|Texas Instruments Incorporated
|IWR1843 Single-Chip 60- to 64-GHz mmWave Sensor
[IBIS Ver]   4.1
[File name]   iwr1843.ibs
[Date]   10/12/2018
[File Rev]   1.0
[Source]
| Texas Instruments Incorporated.
| Analog-eLab Design Center, HPA
| 12500 TI Blvd
| Dallas, TX -75243
[Notes]   Revision History:
| Rev 1.0: 10/12/2018
| - Initial version of the model
| - C_comp although listed in numerical order of value are
|   obtained from varying PVT conditions. For PVT conditions for
|   each specific value refer the buffer description under
|   respective [Model]. IBIS model user is responsible for using
|   appropriate C_comp to simulate for Signal Integrity.
| Rev 1.1  9/9/2019
|  - Added missing package model keyword
|  - Removed redundant references
[Disclaimer]
| This model is designed as an aid for customers of Texas Instruments.
| TI and its licensors and suppliers make no warranties, either expressed
| or implied, with respect to this  model, including the warranties of
| merchantability or fitness for a particular purpose. The model is
| provided solely on an "as is" basis. The entire risk as to its quality
| and performance is with the customer.
| This model is subject to change without notice. Texas Instruments
| Incorporated is not responsible for updating this model.
[Copyright]
(C) Copyright 2018 Texas Instruments Incorporated.All rights reserved.
|  Component IWR1843QGABL
[Component]   IWR1843QGABL
[Manufacturer]   Texas Instruments
[Package]   |161 FCBGA -ABL0161 package
|  variable   typ   min   max
R_pkg   0.05   0.04   0.06
L_pkg   1.0nH   0.8nH   1.2nH
C_pkg   0.2pF   0.16pF   0.24pF
[Pin]   signal_name   model_name   R_pin   L_pin   C_pin
 A1   VSSA   GND   NA   NA   NA
 A2   VOUT_PA   NC   NA   NA   NA
 A3   VSSA   GND   NA   NA   NA
 A5   VSSA   GND   NA   NA   NA
 A7   VSSA   GND   NA   NA   NA
 A9   VSSA   GND   NA   NA   NA
 A10   VOUT_14APLL   NC   NA   NA   NA
 A13   VSSA   GND   NA   NA   NA
 A14   OSC_CLKOUT   NC   NA   NA   NA
 A15   VSSA   GND   NA   NA   NA
 B1   VSSA   GND   NA   NA   NA
 B2   VOUT_PA   NC   NA   NA   NA
 B3   VSSA   GND   NA   NA   NA
 B4   TX1   NC   NA   NA   NA
 B5   VSSA   GND   NA   NA   NA
 B6   TX2   NC   NA   NA   NA
 B7   VSSA   GND   NA   NA   NA
 B8   TX3   NC   NA   NA   NA
 B9   VSSA   GND   NA   NA   NA
 B10   VBGAP   NC   NA   NA   NA
 B11   VIN_18CLK   POWER   NA   NA   NA
 B12   VIN_18VCO   POWER   NA   NA   NA
 B13   VOUT_14SYNTH   NC   NA   NA   NA
 B14   VSSA   GND   NA   NA   NA
 B15   CLKP   NC   NA   NA   NA
 C1   VSSA   GND   NA   NA   NA
 C2   VIN_13RF2   POWER   NA   NA   NA
 C3   VSSA   GND   NA   NA   NA
 C4   VSSA   GND   NA   NA   NA
 C5   VSSA   GND   NA   NA   NA
 C6   VSSA   GND   NA   NA   NA
 C7   VSSA   GND   NA   NA   NA
 C8   VSSA   GND   NA   NA   NA
 C9   VSSA   GND   NA   NA   NA
 C13   GPADC5   NC   NA   NA   NA
 C14   VSSA   GND   NA   NA   NA
 C15   CLKM   NC   NA   NA   NA
 D2   VIN_13RF2   POWER   NA   NA   NA
 D13   SPIA_MOSI   IO1   NA   NA   NA
 D14   GPADC6   NC   NA   NA   NA
 D15   VIOIN_18DIFF   POWER   NA   NA   NA
 E1   VSSA   GND   NA   NA   NA
 E2   VSSA   GND   NA   NA   NA
 E3   VSSA   GND   NA   NA   NA
 E5   VSS   GND   NA   NA   NA
 E6   VSS   GND   NA   NA   NA
 E8   VSS   GND   NA   NA   NA
 E10   VSS   GND   NA   NA   NA
 E11   VSS   GND   NA   NA   NA
 E13   SPIA_CLK   IO1   NA   NA   NA
 E14   SPIA_MISO   IO1   NA   NA   NA
 E15   SPIA_CS_N   IO1   NA   NA   NA
 F2   RX4   NC   NA   NA   NA
 F3   VSSA   GND   NA   NA   NA
 F5   VIN_18BB   POWER   NA   NA   NA
 F9   VSS   GND   NA   NA   NA
 F11   VSS   GND   NA   NA   NA
 F13   SPIB_MOSI   IO1   NA   NA   NA
 F14   SPIB_CLK   IO1   NA   NA   NA
 F15   VIOIN   POWER   NA   NA   NA
 G1   VSSA   GND   NA   NA   NA
 G2   VSSA   GND   NA   NA   NA
 G3   VSSA   GND   NA   NA   NA
 G5   VIN_13RF1   POWER   NA   NA   NA
 G6   VSS   GND   NA   NA   NA
 G7   VSS   GND   NA   NA   NA
 G8   VSS   GND   NA   NA   NA
 G10   VSS   GND   NA   NA   NA
 G13   SYNC_OUT   IO2   NA   NA   NA
 G14   SPIB_MISO   IO1   NA   NA   NA
 G15   VIN_SRAM   POWER   NA   NA   NA
 H2   RX3   NC   NA   NA   NA
 H3   VSSA   GND   NA   NA   NA
 H5   VIN_13RF1   POWER   NA   NA   NA
 H7   VSS   GND   NA   NA   NA
 H9   VSS   GND   NA   NA   NA
 H11   VSS   GND   NA   NA   NA
 H13   GPIO_0   IO1   NA   NA   NA
 H14   SPIB_CS_N   IO1   NA   NA   NA
 H15   VDDIN   POWER   NA   NA   NA
 J1   VSSA   GND   NA   NA   NA
 J2   VSSA   GND   NA   NA   NA
 J3   VSSA   GND   NA   NA   NA
 J5   VIN_13RF1   POWER   NA   NA   NA
 J6   VSS   GND   NA   NA   NA
 J7   VSS   GND   NA   NA   NA
 J8   VSS   GND   NA   NA   NA
 J10   VSS   GND   NA   NA   NA
 J13   GPIO_1   IO1   NA   NA   NA
 J14   LVDS_TXP[0]   ODF   NA   NA   NA
 J15   LVDS_TXM[0]   ODF   NA   NA   NA
 K2   RX2   NC   NA   NA   NA
 K3   VSSA   GND   NA   NA   NA
 K5   VIN_18BB   POWER   NA   NA   NA
 K7   VSS   GND   NA   NA   NA
 K8   VSS   GND   NA   NA   NA
 K9   VSS   GND   NA   NA   NA
 K10   VSS   GND   NA   NA   NA
 K11   VSS   GND   NA   NA   NA
 K13   GPIO_2   IO2   NA   NA   NA
 K14   LVDS_TXP[1]   ODF   NA   NA   NA
 K15   LVDS_TXM[1]   ODF   NA   NA   NA
 L1   VSSA   GND   NA   NA   NA
 L2   VSSA   GND   NA   NA   NA
 L3   VSSA   GND   NA   NA   NA
 L5   VSS   GND   NA   NA   NA
 L6   VSS   GND   NA   NA   NA
 L8   VSS   GND   NA   NA   NA
 L10   VSS   GND   NA   NA   NA
 L13   VPP   POWER   NA   NA   NA
 L14   LVDS_CLKP   ODF   NA   NA   NA
 L15   LVDS_CLKM   ODF   NA   NA   NA
 M2   RX1   NC   NA   NA   NA
 M3   VSSA   GND   NA   NA   NA
 M14   LVDS_FRCLKP   ODF   NA   NA   NA
 M15   LVDS_FRCLKM   ODF   NA   NA   NA
 N1   VSSA   GND   NA   NA   NA
 N2   VSSA   GND   NA   NA   NA
 N3   VSSA   GND   NA   NA   NA
 N4   RS232_RX   IO1   NA   NA   NA
 N5   RS232_TX   IO1   NA   NA   NA
 N6   NERROR_OUT   IOOD   NA   NA   NA
 N7   NERROR_IN   IOOD   NA   NA   NA
 N8   MCU_CLKOUT   IO1   NA   NA   NA
 N9   WARM_RESET   IOOD   NA   NA   NA
 N10   TMS   IO2   NA   NA   NA
 N11   VDDIN   POWER   NA   NA   NA
 N12   QSPI[1]   IO1   NA   NA   NA
 N13   TDO   IO2   NA   NA   NA
 N14   DMM_SYNC   IO1   NA   NA   NA
 N15   GPIO_47   IO1   NA   NA   NA
 P1   GPADC1   NC   NA   NA   NA
 P2   GPADC2   NC   NA   NA   NA
 P3   GPADC3   NC   NA   NA   NA
 P4   SYNC_IN   IO2   NA   NA   NA
 P5   GPIO_32   IO1   NA   NA   NA
 P6   GPIO_34   IO1   NA   NA   NA
 P7   GPIO_36   IO1   NA   NA   NA
 P8   GPIO_38   IO1   NA   NA   NA
 P9   PMIC_CLKOUT   IO2   NA   NA   NA
 P10   TCK   IO2   NA   NA   NA
 P11   QSPI_CS_N   IO1   NA   NA   NA
 P12   QSPI[3]   IO1   NA   NA   NA
 P13   SPI_HOST_INTR   NC   NA   NA   NA
 P14   VNWA   POWER   NA   NA   NA
 P15   VDDIN   POWER   NA   NA   NA
 R1   VSSA   GND   NA   NA   NA
 R2   GPADC4   NC   NA   NA   NA
 R3   NRESET   NC   NA   NA   NA
 R4   GPIO_31   IO1   NA   NA   NA
 R5   GPIO_33   IO1   NA   NA   NA
 R6   VDDIN   POWER   NA   NA   NA
 R7   GPIO_35   IO1   NA   NA   NA
 R8   GPIO_37   IO1   NA   NA   NA
 R9   VIOIN_18   POWER   NA   NA   NA
 R10   VIOIN   POWER   NA   NA   NA
 R11   TDI   IO2   NA   NA   NA
 R12   QSPI_CLK   IO1   NA   NA   NA
 R13   QSPI[0]   IO2   NA   NA   NA
 R14   QSPI[2]   IO2   NA   NA   NA
 R15   VSS   GND   NA   NA   NA
[Diff Pin]  inv_pin  vdiff  tdelay_typ  tdelay_min  tdelay_max
   J14   J15   0.1   NA   NA   NA
   K14   K15   0.1   NA   NA   NA
   L14   L15   0.1   NA   NA   NA
   M14   M15   0.1   NA   NA   NA
[Package Model]  IWR1843QGABL
| Model IOOD
[Model Selector] IOOD
|SC1 IS A SLEW RATE CONTROL PIN
|5% SUPPLY VARIATION MODES WITH 1.8V NOM SUPPLY
IOOD_V_PUPDOFF_5P_SC1_1P8  Cell operated at 1.8(nom)
|IOOD_V_PUPDOFF_5P_SC1_1P8; BUFFER WITH WEAK PULUP/PULLDOWN OFF AT 5% SUPPLY
|VARIATION WITH SC1=1 MEANING SLOW MODE OF OPERATION
IOOD_V_PD_ON_5P_!SC1_1P8  Cell operated at 1.8(nom)
|IOOD_V_PD_ON_5P_!SC1_1P8; BUFFER WITH WEAK_PULLDOWN_ON AT 5% SUPPLY
|VARIATION WITH SC1=0 MEANING FAST MODE OF OPERATION
IOOD_V_PD_ON_5P_SC1_1P8  Cell operated at 1.8(nom)
|IOOD_V_PD_ON_5P_SC1_1P8; BUFFER WITH WEAK_PULLDOWN_ON AT 5% SUPPLY
|VARIATION WITH SC1=1 MEANING SLOW MODE OF OPERATION
IOOD_V_PU_ON_5P_!SC1_1P8  Cell operated at 1.8(nom)
|IOOD_V_PU_ON_5P_!SC1_1P8; BUFFER WITH WEAK_PULLUP_ON AT 5% SUPPLY
|VARIATION WITH SC1=0 MEANING FAST MODE OF OPERATION
IOOD_V_PUPDOFF_5P_!SC1_1P8  Cell operated at 1.8(nom)
|IOOD_V_PUPDOFF_5P_!SC1_1P8; BUFFER WITH WEAK PULUP/PULLDOWN OFF AT 5% SUPPLY
|VARIATION WITH SC1=0 MEANING FAST MODE OF OPERATION
IOOD_V_PU_ON_5P_SC1_1P8  Cell operated at 1.8(nom)
|IOOD_V_PU_ON_5P_SC1_1P8; BUFFER WITH WEAK_PULLUP_ON AT 5% SUPPLY
|VARIATION WITH SC1=1 MEANING SLOW MODE OF OPERATION
|5% SUPPLY VARIATION MODES WITH 3.3V NOM SUPPLY
IOOD_V_PUPDOFF_5P_SC1_3P3  Cell operated at 3.3(nom)
|IOOD_V_PUPDOFF_5P_SC1_3P3; BUFFER WITH WEAK PULUP/PULLDOWN OFF AT 5% SUPPLY
|VARIATION WITH SC1=1 MEANING SLOW MODE OF OPERATION
IOOD_V_PD_ON_5P_!SC1_3P3  Cell operated at 3.3(nom)
|IOOD_V_PD_ON_5P_!SC1_3P3; BUFFER WITH WEAK_PULLDOWN_ON AT 5% SUPPLY
|VARIATION WITH SC1=0 MEANING FAST MODE OF OPERATION
IOOD_V_PD_ON_5P_SC1_3P3  Cell operated at 3.3(nom)
|IOOD_V_PD_ON_5P_SC1_3P3; BUFFER WITH WEAK_PULLDOWN_ON AT 5% SUPPLY
|VARIATION WITH SC1=1 MEANING SLOW MODE OF OPERATION
IOOD_V_PU_ON_5P_!SC1_3P3  Cell operated at 3.3(nom)
|IOOD_V_PU_ON_5P_!SC1_3P3; BUFFER WITH WEAK_PULLUP_ON AT 5% SUPPLY
|VARIATION WITH SC1=0 MEANING FAST MODE OF OPERATION
IOOD_V_PUPDOFF_5P_!SC1_3P3  Cell operated at 3.3(nom)
|IOOD_V_PUPDOFF_5P_!SC1_3P3; BUFFER WITH WEAK PULUP/PULLDOWN OFF AT 5% SUPPLY
|VARIATION WITH SC1=0 MEANING FAST MODE OF OPERATION
IOOD_V_PU_ON_5P_SC1_3P3  Cell operated at 3.3(nom)
|IOOD_V_PU_ON_5P_SC1_3P3; BUFFER WITH WEAK_PULLUP_ON AT 5% SUPPLY
|VARIATION WITH SC1=1 MEANING SLOW MODE OF OPERATION
| 10% SUPPLY VARIATION MODES WITH 1.8V NOM SUPPLY
IOOD_V_PUPDOFF_10P_SC1_1P8  Cell operated at 1.8(nom)
|IOOD_V_PUPDOFF_10P_SC1_1P8; BUFFER WITH WEAK PULUP/PULLDOWN OFF AT 10% SUPPLY
|VARIATION WITH SC1=1 MEANING SLOW MODE OF OPERATION
IOOD_V_PD_ON_10P_!SC1_1P8  Cell operated at 1.8(nom)
|IOOD_V_PD_ON_10P_!SC1_1P8; BUFFER WITH WEAK_PULLDOWN_ON AT 10% SUPPLY
|VARIATION WITH SC1=0 MEANING FAST MODE OF OPERATION
IOOD_V_PD_ON_10P_SC1_1P8  Cell operated at 1.8(nom)
|IOOD_V_PD_ON_10P_SC1_1P8; BUFFER WITH WEAK_PULLDOWN_ON AT 10% SUPPLY
|VARIATION WITH SC1=1 MEANING SLOW MODE OF OPERATION
IOOD_V_PU_ON_10P_!SC1_1P8  Cell operated at 1.8(nom)
|IOOD_V_PU_ON_10P_!SC1_1P8; BUFFER WITH WEAK_PULLUP_ON AT 10% SUPPLY
|VARIATION WITH SC1=0 MEANING FAST MODE OF OPERATION
IOOD_V_PUPDOFF_10P_!SC1_1P8  Cell operated at 1.8(nom)
|IOOD_V_PUPDOFF_10P_!SC1_1P8; BUFFER WITH WEAK PULUP/PULLDOWN OFF AT 10% SUPPLY
|VARIATION WITH SC1=0 MEANING FAST MODE OF OPERATION
IOOD_V_PU_ON_10P_SC1_1P8  Cell operated at 1.8(nom)
|IOOD_V_PU_ON_10P_SC1_1P8; BUFFER WITH WEAK_PULLUP_ON AT 10% SUPPLY
|VARIATION WITH SC1=1 MEANING SLOW MODE OF OPERATION
| 10% SUPPLY VARIATION MODES WITH 3.3V NOM SUPPLY
IOOD_V_PUPDOFF_10P_SC1_3P3  Cell operated at 3.3(nom)
|IOOD_V_PUPDOFF_10P_SC1_3P3; BUFFER WITH WEAK PULUP/PULLDOWN OFF AT 10% SUPPLY
|VARIATION WITH SC1=1 MEANING SLOW MODE OF OPERATION
IOOD_V_PD_ON_10P_!SC1_3P3  Cell operated at 3.3(nom)
|IOOD_V_PD_ON_10P_!SC1_3P3; BUFFER WITH WEAK_PULLDOWN_ON 10% SUPPLY
|VARIATION WITH SC1=0 MEANING FAST MODE OF OPERATION
IOOD_V_PD_ON_10P_SC1_3P3  Cell operated at 3.3(nom)
|IOOD_V_PD_ON_10P_SC1_3P3; BUFFER WITH WEAK_PULLDOWN_ON AT 10% SUPPLY
|VARIATION WITH SC1=1 MEANING SLOW MODE OF OPERATION
IOOD_V_PU_ON_10P_!SC1_3P3  Cell operated at 3.3(nom)
|IOOD_V_PU_ON_10P_!SC1_3P3; BUFFER WITH WEAK_PULLUP_ON AT 10% SUPPLY
|VARIATION WITH SC1=0 MEANING FAST MODE OF OPERATION
IOOD_V_PUPDOFF_10P_!SC1_3P3  Cell operated at 3.3(nom)
|IOOD_V_PUPDOFF_10P_!SC1_3P3; BUFFER WITH WEAK PULUP/PULLDOWN OFF AT 10% SUPPLY
|VARIATION WITH SC1=0 MEANING FAST MODE OF OPERATION
IOOD_V_PU_ON_10P_SC1_3P3  Cell operated at 3.3(nom)
|IOOD_V_PU_ON_10P_SC1_3P3; BUFFER WITH WEAK_PULLUP_ON AT 10% SUPPLY
|VARIATION WITH SC1=1 MEANING SLOW MODE OF OPERATION
| Model IO1
[Model Selector] IO1
|SC1 IS A SLEW RATE CONTROL PIN
|5% SUPPLY VARIATION MODES WITH 1.8V NOM SUPPLY
IO1_V_PUPDOFF_5P_SC1_1P8  Cell operated at 1.8(nom)
|IO1_V_PUPDOFF_5P_SC1_1P8; BUFFER WITH WEAK PULUP/PULLDOWN OFF AT 5% SUPPLY
|VARIATION WITH SC1=1 MEANING SLOW MODE OF OPERATION
IO1_V_PD_ON_5P_!SC1_1P8  Cell operated at 1.8(nom)
|IO1_V_PD_ON_5P_!SC1_1P8; BUFFER WITH WEAK_PULLDOWN_ON AT 5% SUPPLY
|VARIATION WITH SC1=0 MEANING FAST MODE OF OPERATION
IO1_V_PD_ON_5P_SC1_1P8  Cell operated at 1.8(nom)
|IO1_V_PD_ON_5P_SC1_1P8; BUFFER WITH WEAK_PULLDOWN_ON AT 5% SUPPLY
|VARIATION WITH SC1=1 MEANING SLOW MODE OF OPERATION
IO1_V_PU_ON_5P_!SC1_1P8  Cell operated at 1.8(nom)
|IO1_V_PU_ON_5P_!SC1_1P8; BUFFER WITH WEAK_PULLUP_ON AT 5% SUPPLY
|VARIATION WITH SC1=0 MEANING FAST MODE OF OPERATION
IO1_V_PUPDOFF_5P_!SC1_1P8  Cell operated at 1.8(nom)
|IO1_V_PUPDOFF_5P_!SC1_1P8; BUFFER WITH WEAK PULUP/PULLDOWN OFF AT 5% SUPPLY
|VARIATION WITH SC1=0 MEANING FAST MODE OF OPERATION
IO1_V_PU_ON_5P_SC1_1P8  Cell operated at 1.8(nom)
|IO1_V_PU_ON_5P_SC1_1P8; BUFFER WITH WEAK_PULLUP_ON AT 5% SUPPLY
|VARIATION WITH SC1=1 MEANING SLOW MODE OF OPERATION
|5% SUPPLY VARIATION MODES WITH 3.3V NOM SUPPLY
IO1_V_PUPDOFF_5P_SC1_3P3  Cell operated at 3.3(nom)
|IO1_V_PUPDOFF_5P_SC1_3P3; BUFFER WITH WEAK PULUP/PULLDOWN OFF AT 5% SUPPLY
|VARIATION WITH SC1=1 MEANING SLOW MODE OF OPERATION
IO1_V_PD_ON_5P_!SC1_3P3  Cell operated at 3.3(nom)
|IO1_V_PD_ON_5P_!SC1_3P3; BUFFER WITH WEAK_PULLDOWN_ON AT 5% SUPPLY
|VARIATION WITH SC1=0 MEANING FAST MODE OF OPERATION
IO1_V_PD_ON_5P_SC1_3P3  Cell operated at 3.3(nom)
|IO1_V_PD_ON_5P_SC1_3P3; BUFFER WITH WEAK_PULLDOWN_ON AT 5% SUPPLY
|VARIATION WITH SC1=1 MEANING SLOW MODE OF OPERATION
IO1_V_PU_ON_5P_!SC1_3P3  Cell operated at 3.3(nom)
|IO1_V_PU_ON_5P_!SC1_3P3; BUFFER WITH WEAK_PULLUP_ON AT 5% SUPPLY
|VARIATION WITH SC1=0 MEANING FAST MODE OF OPERATION
IO1_V_PUPDOFF_5P_!SC1_3P3  Cell operated at 3.3(nom)
|IO1_V_PUPDOFF_5P_!SC1_3P3; BUFFER WITH WEAK PULUP/PULLDOWN OFF AT 5% SUPPLY
|VARIATION WITH SC1=0 MEANING FAST MODE OF OPERATION
IO1_V_PU_ON_5P_SC1_3P3  Cell operated at 3.3(nom)
|IO1_V_PU_ON_5P_SC1_3P3; BUFFER WITH WEAK_PULLUP_ON AT 5% SUPPLY
|VARIATION WITH SC1=1 MEANING SLOW MODE OF OPERATION
| 10% SUPPLY VARIATION MODES WITH 1.8V NOM SUPPLY
IO1_V_PUPDOFF_10P_SC1_1P8  Cell operated at 1.8(nom)
|IO1_V_PUPDOFF_10P_SC1_1P8; BUFFER WITH WEAK PULUP/PULLDOWN OFF AT 10% SUPPLY
|VARIATION WITH SC1=1 MEANING SLOW MODE OF OPERATION
IO1_V_PD_ON_10P_!SC1_1P8  Cell operated at 1.8(nom)
|IO1_V_PD_ON_10P_!SC1_1P8; BUFFER WITH WEAK_PULLDOWN_ON AT 10% SUPPLY
|VARIATION WITH SC1=0 MEANING FAST MODE OF OPERATION
IO1_V_PD_ON_10P_SC1_1P8  Cell operated at 1.8(nom)
|IO1_V_PD_ON_10P_SC1_1P8; BUFFER WITH WEAK_PULLDOWN_ON AT 10% SUPPLY
|VARIATION WITH SC1=1 MEANING SLOW MODE OF OPERATION
IO1_V_PU_ON_10P_!SC1_1P8  Cell operated at 1.8(nom)
|IO1_V_PU_ON_10P_!SC1_1P8; BUFFER WITH WEAK_PULLUP_ON AT 10% SUPPLY
|VARIATION WITH SC1=0 MEANING FAST MODE OF OPERATION
IO1_V_PUPDOFF_10P_!SC1_1P8  Cell operated at 1.8(nom)
|IO1_V_PUPDOFF_10P_!SC1_1P8; BUFFER WITH WEAK PULUP/PULLDOWN OFF AT 10% SUPPLY
|VARIATION WITH SC1=0 MEANING FAST MODE OF OPERATION
IO1_V_PU_ON_10P_SC1_1P8  Cell operated at 1.8(nom)
|IO1_V_PU_ON_10P_SC1_1P8; BUFFER WITH WEAK_PULLUP_ON AT 10% SUPPLY
|VARIATION WITH SC1=1 MEANING SLOW MODE OF OPERATION
| 10% SUPPLY VARIATION MODES WITH 3.3V NOM SUPPLY
IO1_V_PUPDOFF_10P_SC1_3P3  Cell operated at 3.3(nom)
|IO1_V_PUPDOFF_10P_SC1_3P3; BUFFER WITH WEAK PULUP/PULLDOWN OFF AT 10% SUPPLY
|VARIATION WITH SC1=1 MEANING SLOW MODE OF OPERATION
IO1_V_PD_ON_10P_!SC1_3P3  Cell operated at 3.3(nom)
|IO1_V_PD_ON_10P_!SC1_3P3; BUFFER WITH WEAK_PULLDOWN_ON 10% SUPPLY
|VARIATION WITH SC1=0 MEANING FAST MODE OF OPERATION
IO1_V_PD_ON_10P_SC1_3P3  Cell operated at 3.3(nom)
|IO1_V_PD_ON_10P_SC1_3P3; BUFFER WITH WEAK_PULLDOWN_ON AT 10% SUPPLY
|VARIATION WITH SC1=1 MEANING SLOW MODE OF OPERATION
IO1_V_PU_ON_10P_!SC1_3P3  Cell operated at 3.3(nom)
|IO1_V_PU_ON_10P_!SC1_3P3; BUFFER WITH WEAK_PULLUP_ON AT 10% SUPPLY
|VARIATION WITH SC1=0 MEANING FAST MODE OF OPERATION
IO1_V_PUPDOFF_10P_!SC1_3P3  Cell operated at 3.3(nom)
|IO1_V_PUPDOFF_10P_!SC1_3P3; BUFFER WITH WEAK PULUP/PULLDOWN OFF AT 10% SUPPLY
|VARIATION WITH SC1=0 MEANING FAST MODE OF OPERATION
IO1_V_PU_ON_10P_SC1_3P3  Cell operated at 3.3(nom)
|IO1_V_PU_ON_10P_SC1_3P3; BUFFER WITH WEAK_PULLUP_ON AT 10% SUPPLY
|VARIATION WITH SC1=1 MEANING SLOW MODE OF OPERATION
| Model IO2
[Model Selector] IO2
|SC1 IS A SLEW RATE CONTROL PIN
|5% SUPPLY VARIATION MODES WITH 1.8V NOM SUPPLY
IO2_H_PUPDOFF_5P_SC1_1P8  Cell operated at 1.8(nom)
|IO2_H_PUPDOFF_5P_SC1_1P8; BUFFER WITH WEAK PULUP/PULLDOWN OFF AT 5% SUPPLY
|VARIATION WITH SC1=1 MEANING SLOW MODE OF OPERATION
IO2_H_PD_ON_5P_!SC1_1P8  Cell operated at 1.8(nom)
|IO2_H_PD_ON_5P_!SC1_1P8; BUFFER WITH WEAK_PULLDOWN_ON AT 5% SUPPLY
|VARIATION WITH SC1=0 MEANING FAST MODE OF OPERATION
IO2_H_PD_ON_5P_SC1_1P8  Cell operated at 1.8(nom)
|IO2_H_PD_ON_5P_SC1_1P8; BUFFER WITH WEAK_PULLDOWN_ON AT 5% SUPPLY
|VARIATION WITH SC1=1 MEANING SLOW MODE OF OPERATION
IO2_H_PU_ON_5P_!SC1_1P8  Cell operated at 1.8(nom)
|IO2_H_PU_ON_5P_!SC1_1P8; BUFFER WITH WEAK_PULLUP_ON AT 5% SUPPLY
|VARIATION WITH SC1=0 MEANING FAST MODE OF OPERATION
IO2_H_PUPDOFF_5P_!SC1_1P8  Cell operated at 1.8(nom)
|IO2_H_PUPDOFF_5P_!SC1_1P8; BUFFER WITH WEAK PULUP/PULLDOWN OFF AT 5% SUPPLY
|VARIATION WITH SC1=0 MEANING FAST MODE OF OPERATION
IO2_H_PU_ON_5P_SC1_1P8  Cell operated at 1.8(nom)
|IO2_H_PU_ON_5P_SC1_1P8; BUFFER WITH WEAK_PULLUP_ON AT 5% SUPPLY
|VARIATION WITH SC1=1 MEANING SLOW MODE OF OPERATION
|5% SUPPLY VARIATION MODES WITH 3.3V NOM SUPPLY
IO2_H_PUPDOFF_5P_SC1_3P3  Cell operated at 3.3(nom)
|IO2_H_PUPDOFF_5P_SC1_3P3; BUFFER WITH WEAK PULUP/PULLDOWN OFF AT 5% SUPPLY
|VARIATION WITH SC1=1 MEANING SLOW MODE OF OPERATION
IO2_H_PD_ON_5P_!SC1_3P3  Cell operated at 3.3(nom)
|IO2_H_PD_ON_5P_!SC1_3P3; BUFFER WITH WEAK_PULLDOWN_ON AT 5% SUPPLY
|VARIATION WITH SC1=0 MEANING FAST MODE OF OPERATION
IO2_H_PD_ON_5P_SC1_3P3  Cell operated at 3.3(nom)
|IO2_H_PD_ON_5P_SC1_3P3; BUFFER WITH WEAK_PULLDOWN_ON AT 5% SUPPLY
|VARIATION WITH SC1=1 MEANING SLOW MODE OF OPERATION
IO2_H_PU_ON_5P_!SC1_3P3  Cell operated at 3.3(nom)
|IO2_H_PU_ON_5P_!SC1_3P3; BUFFER WITH WEAK_PULLUP_ON AT 5% SUPPLY
|VARIATION WITH SC1=0 MEANING FAST MODE OF OPERATION
IO2_H_PUPDOFF_5P_!SC1_3P3  Cell operated at 3.3(nom)
|IO2_H_PUPDOFF_5P_!SC1_3P3; BUFFER WITH WEAK PULUP/PULLDOWN OFF AT 5% SUPPLY
|VARIATION WITH SC1=0 MEANING FAST MODE OF OPERATION
IO2_H_PU_ON_5P_SC1_3P3  Cell operated at 3.3(nom)
|IO2_H_PU_ON_5P_SC1_3P3; BUFFER WITH WEAK_PULLUP_ON AT 5% SUPPLY
|VARIATION WITH SC1=1 MEANING SLOW MODE OF OPERATION
| 10% SUPPLY VARIATION MODES WITH 1.8V NOM SUPPLY
IO2_H_PUPDOFF_10P_SC1_1P8  Cell operated at 1.8(nom)
|IO2_H_PUPDOFF_10P_SC1_1P8; BUFFER WITH WEAK PULUP/PULLDOWN OFF AT 10% SUPPLY
|VARIATION WITH SC1=1 MEANING SLOW MODE OF OPERATION
IO2_H_PD_ON_10P_!SC1_1P8  Cell operated at 1.8(nom)
|IO2_H_PD_ON_10P_!SC1_1P8; BUFFER WITH WEAK_PULLDOWN_ON AT 10% SUPPLY
|VARIATION WITH SC1=0 MEANING FAST MODE OF OPERATION
IO2_H_PD_ON_10P_SC1_1P8  Cell operated at 1.8(nom)
|IO2_H_PD_ON_10P_SC1_1P8; BUFFER WITH WEAK_PULLDOWN_ON AT 10% SUPPLY
|VARIATION WITH SC1=1 MEANING SLOW MODE OF OPERATION
IO2_H_PU_ON_10P_!SC1_1P8  Cell operated at 1.8(nom)
|IO2_H_PU_ON_10P_!SC1_1P8; BUFFER WITH WEAK_PULLUP_ON AT 10% SUPPLY
|VARIATION WITH SC1=0 MEANING FAST MODE OF OPERATION
IO2_H_PUPDOFF_10P_!SC1_1P8  Cell operated at 1.8(nom)
|IO2_H_PUPDOFF_10P_!SC1_1P8; BUFFER WITH WEAK PULUP/PULLDOWN OFF AT 10% SUPPLY
|VARIATION WITH SC1=0 MEANING FAST MODE OF OPERATION
IO2_H_PU_ON_10P_SC1_1P8  Cell operated at 1.8(nom)
|IO2_H_PU_ON_10P_SC1_1P8; BUFFER WITH WEAK_PULLUP_ON AT 10% SUPPLY
|VARIATION WITH SC1=1 MEANING SLOW MODE OF OPERATION
| 10% SUPPLY VARIATION MODES WITH 3.3V NOM SUPPLY
IO2_H_PUPDOFF_10P_SC1_3P3  Cell operated at 3.3(nom)
|IO2_H_PUPDOFF_10P_SC1_3P3; BUFFER WITH WEAK PULUP/PULLDOWN OFF AT 10% SUPPLY
|VARIATION WITH SC1=1 MEANING SLOW MODE OF OPERATION
IO2_H_PD_ON_10P_!SC1_3P3  Cell operated at 3.3(nom)
|IO2_H_PD_ON_10P_!SC1_3P3; BUFFER WITH WEAK_PULLDOWN_ON 10% SUPPLY
|VARIATION WITH SC1=0 MEANING FAST MODE OF OPERATION
IO2_H_PD_ON_10P_SC1_3P3  Cell operated at 3.3(nom)
|IO2_H_PD_ON_10P_SC1_3P3; BUFFER WITH WEAK_PULLDOWN_ON AT 10% SUPPLY
|VARIATION WITH SC1=1 MEANING SLOW MODE OF OPERATION
IO2_H_PU_ON_10P_!SC1_3P3  Cell operated at 3.3(nom)
|IO2_H_PU_ON_10P_!SC1_3P3; BUFFER WITH WEAK_PULLUP_ON AT 10% SUPPLY
|VARIATION WITH SC1=0 MEANING FAST MODE OF OPERATION
IO2_H_PUPDOFF_10P_!SC1_3P3  Cell operated at 3.3(nom)
|IO2_H_PUPDOFF_10P_!SC1_3P3; BUFFER WITH WEAK PULUP/PULLDOWN OFF AT 10% SUPPLY
|VARIATION WITH SC1=0 MEANING FAST MODE OF OPERATION
IO2_H_PU_ON_10P_SC1_3P3  Cell operated at 3.3(nom)
|IO2_H_PU_ON_10P_SC1_3P3; BUFFER WITH WEAK_PULLUP_ON AT 10% SUPPLY
|VARIATION WITH SC1=1 MEANING SLOW MODE OF OPERATION
| Model ODF
[Model Selector] ODF
ODF_MODE_10P_1P8  Cell operated at 1.8(nom)
|ODF_MODE_10P_1P8; LVDS DRIVER MODE WITH 10PER VDDS
ODF_MODE_5P_1P8  Cell operated at 1.8(nom)
[Define Package Model]   IWR1843QGABL
[Manufacturer]   TI
[OEM]   TI
[Description]   xwr1843 package
|[Number of Sections]   1
[Number of Pins]   82
[Pin Numbers]
|[Pin Name]  Net Number   Net Name   Net's All Pins
R6   | 1   VDDIN   R6
   |P15
   |H15
   |N11
C15   | 2   CLKM   C15
B15   | 3   CLKP   B15
N15   | 4   DMM_CLK   N15
N14   | 5   DMM_SYNC   N14
R4   | 6   DP0   R4
P5   | 7   DP1   P5
R5   | 8   DP2   R5
P6   | 9   DP3   P6
R7   | 10   DP4   R7
P7   | 11   DP5   P7
R8   | 12   DP6   R8
P8   | 13   DP7   P8
P1   | 14   GPADC_1   P1
P2   | 15   GPADC_2   P2
P3   | 16   GPADC_3   P3
R2   | 17   GPADC_4   R2
C13   | 18   GPADC_5   C13
D14   | 19   GPADC_6   D14
H13   | 20   GPIO[0]   H13
J13   | 21   GPIO[1]   J13
K13   | 22   GPIO[2]   K13
L15   | 23   LVDS_CLKM   L15
L14   | 24   LVDS_CLKP   L14
M15   | 25   LVDS_FRCLKM   M15
M14   | 26   LVDS_FRCLKP   M14
J15   | 27   LVDS_TXM[0]   J15
K15   | 28   LVDS_TXM[1]   K15
J14   | 29   LVDS_TXP[0]   J14
K14   | 30   LVDS_TXP[1]   K14
N8   | 31   MCU_CLKOUT   N8
E14   | 32   MISO_1   E14
G14   | 33   MISO_2   G14
D13   | 34   MOSI_1   D13
F13   | 35   MOSI_2   F13
N7   | 36   NERROR_IN   N7
N6   | 37   NERROR_OUT   N6
R3   | 38   NRESET   R3
A14   | 39   OSC_CLKOUT   A14
P9   | 40   PMIC_CLKOUT   P9
R13   | 41   QSPI[0]   R13
N12   | 42   QSPI[1]   N12
R14   | 43   QSPI[2]   R14
P12   | 44   QSPI[3]   P12
R12   | 45   QSPI_CLK   R12
P11   | 46   QSPI_CS   P11
N4   | 47   RS232_RX   N4
N5   | 48   RS232_TX   N5
M2   | 49   RX1   M2
K2   | 50   RX2   K2
H2   | 51   RX3   H2
F2   | 52   RX4   F2
E13   | 53   SPI_CLK_1   E13
F14   | 54   SPI_CLK_2   F14
E15   | 55   SPI_CS_1   E15
H14   | 56   SPI_CS_2   H14
P13   | 57   SPI_HOST_INTR_1   P13
P4   | 58   SYNC_IN   P4
G13   | 59   SYNC_OUT   G13
P10   | 60   TCK   P10
R11   | 61   TDI   R11
N13   | 62   TDO   N13
N10   | 63   TMS   N10
B4   | 64   TX1   B4
B6   | 65   TX2   B6
B8   | 66   TX3   B8
B10   | 67   VBGAP   B10
J5   | 68   VIN_13RF1   J5
   |H5
   |G5
D2   | 69   VIN_13RF2   D2
   |C2
K5   | 70   VIN_18BB   K5
   |F5
B11   | 71   VIN_18CLK   B11
B12   | 72   VIN_18VCO   B12
G15   | 73   VIN_SRAM   G15
R10   | 74   VIOIN   R10
   |F15
R9   | 75   VIOIN_18   R9
D15   | 76   VIOIN_18DIFF   D15
P14   | 77   VNWA   P14
A10   | 78   VOUT_14APLL   A10
B13   | 79   VOUT_14SYNTH   B13
B2   | 80   VOUT_PA   B2
   |A2
L13   | 81   VPP   L13
N9   | 82   WARM_RESET   N9
[Model Data]
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[End Model Data]
[End Package Model]
| Models and submodels in the file (74): IOOD_V_PUPDOFF_5P_SC1_1P8 (I/O_open_drain), IOOD_V_PD_ON_5P_!SC1_1P8 (I/O_open_drain), IOOD_V_PD_ON_5P_SC1_1P8 (I/O_open_drain), IOOD_V_PU_ON_5P_!SC1_1P8 (I/O_open_drain), IOOD_V_PUPDOFF_5P_!SC1_1P8 (I/O_open_drain), IOOD_V_PU_ON_5P_SC1_1P8 (I/O_open_drain), IOOD_V_PUPDOFF_5P_SC1_3P3 (I/O_open_drain), IOOD_V_PD_ON_5P_!SC1_3P3 (I/O_open_drain), IOOD_V_PD_ON_5P_SC1_3P3 (I/O_open_drain), IOOD_V_PU_ON_5P_!SC1_3P3 (I/O_open_drain), IOOD_V_PUPDOFF_5P_!SC1_3P3 (I/O_open_drain), IOOD_V_PU_ON_5P_SC1_3P3 (I/O_open_drain), IOOD_V_PUPDOFF_10P_SC1_1P8 (I/O_open_drain), IOOD_V_PD_ON_10P_!SC1_1P8 (I/O_open_drain), IOOD_V_PD_ON_10P_SC1_1P8 (I/O_open_drain), IOOD_V_PU_ON_10P_!SC1_1P8 (I/O_open_drain), IOOD_V_PUPDOFF_10P_!SC1_1P8 (I/O_open_drain), IOOD_V_PU_ON_10P_SC1_1P8 (I/O_open_drain), IOOD_V_PUPDOFF_10P_SC1_3P3 (I/O_open_drain), IOOD_V_PD_ON_10P_!SC1_3P3 (I/O_open_drain), IOOD_V_PD_ON_10P_SC1_3P3 (I/O_open_drain), IOOD_V_PU_ON_10P_!SC1_3P3 (I/O_open_drain), IOOD_V_PUPDOFF_10P_!SC1_3P3 (I/O_open_drain), IOOD_V_PU_ON_10P_SC1_3P3 (I/O_open_drain), IO1_V_PUPDOFF_5P_SC1_1P8 (I/O), IO1_V_PD_ON_5P_!SC1_1P8 (I/O), IO1_V_PD_ON_5P_SC1_1P8 (I/O), IO1_V_PU_ON_5P_!SC1_1P8 (I/O), IO1_V_PUPDOFF_5P_!SC1_1P8 (I/O), IO1_V_PU_ON_5P_SC1_1P8 (I/O), IO1_V_PUPDOFF_5P_SC1_3P3 (I/O), IO1_V_PD_ON_5P_!SC1_3P3 (I/O), IO1_V_PD_ON_5P_SC1_3P3 (I/O), IO1_V_PU_ON_5P_!SC1_3P3 (I/O), IO1_V_PUPDOFF_5P_!SC1_3P3 (I/O), IO1_V_PU_ON_5P_SC1_3P3 (I/O), IO1_V_PUPDOFF_10P_SC1_1P8 (I/O), IO1_V_PD_ON_10P_!SC1_1P8 (I/O), IO1_V_PD_ON_10P_SC1_1P8 (I/O), IO1_V_PU_ON_10P_!SC1_1P8 (I/O), IO1_V_PUPDOFF_10P_!SC1_1P8 (I/O), IO1_V_PU_ON_10P_SC1_1P8 (I/O), IO1_V_PUPDOFF_10P_SC1_3P3 (I/O), IO1_V_PD_ON_10P_!SC1_3P3 (I/O), IO1_V_PD_ON_10P_SC1_3P3 (I/O), IO1_V_PU_ON_10P_!SC1_3P3 (I/O), IO1_V_PUPDOFF_10P_!SC1_3P3 (I/O), IO1_V_PU_ON_10P_SC1_3P3 (I/O), IO2_H_PUPDOFF_5P_SC1_1P8 (I/O), IO2_H_PD_ON_5P_!SC1_1P8 (I/O), IO2_H_PD_ON_5P_SC1_1P8 (I/O), IO2_H_PU_ON_5P_!SC1_1P8 (I/O), IO2_H_PUPDOFF_5P_!SC1_1P8 (I/O), IO2_H_PU_ON_5P_SC1_1P8 (I/O), IO2_H_PUPDOFF_5P_SC1_3P3 (I/O), IO2_H_PD_ON_5P_!SC1_3P3 (I/O), IO2_H_PD_ON_5P_SC1_3P3 (I/O), IO2_H_PU_ON_5P_!SC1_3P3 (I/O), IO2_H_PUPDOFF_5P_!SC1_3P3 (I/O), IO2_H_PU_ON_5P_SC1_3P3 (I/O), IO2_H_PUPDOFF_10P_SC1_1P8 (I/O), IO2_H_PD_ON_10P_!SC1_1P8 (I/O), IO2_H_PD_ON_10P_SC1_1P8 (I/O), IO2_H_PU_ON_10P_!SC1_1P8 (I/O), IO2_H_PUPDOFF_10P_!SC1_1P8 (I/O), IO2_H_PU_ON_10P_SC1_1P8 (I/O), IO2_H_PUPDOFF_10P_SC1_3P3 (I/O), IO2_H_PD_ON_10P_!SC1_3P3 (I/O), IO2_H_PD_ON_10P_SC1_3P3 (I/O), IO2_H_PU_ON_10P_!SC1_3P3 (I/O), IO2_H_PUPDOFF_10P_!SC1_3P3 (I/O), IO2_H_PU_ON_10P_SC1_3P3 (I/O), ODF_MODE_10P_1P8 (3-state), ODF_MODE_5P_1P8 (3-state)
